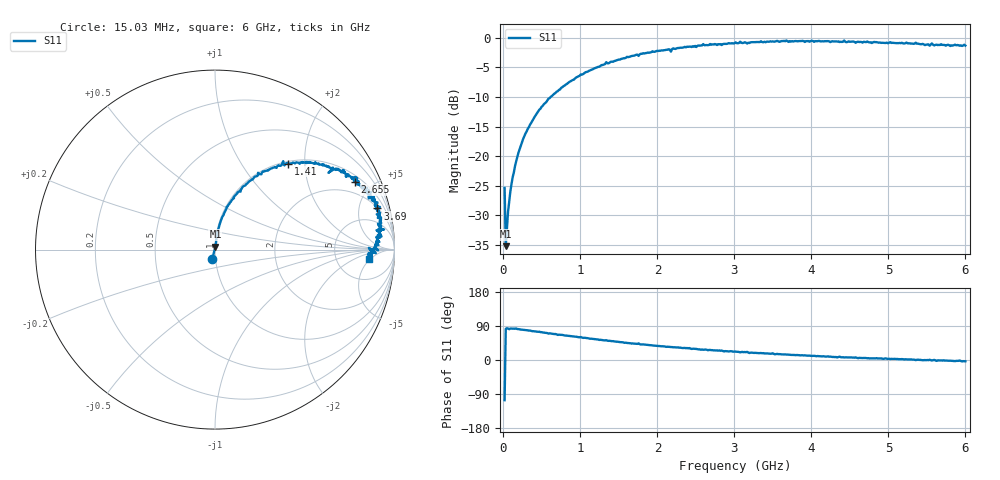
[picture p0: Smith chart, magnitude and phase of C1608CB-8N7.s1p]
!	Network	Analyzer	HP8753E.07.74:	Oct	30	2002	Serial	No.	JP38451487
!	Hewlett-Packard
!	28	Aug	2009	7:51:57
!	Frequency	S11
#	HZ	S	RI	R	50
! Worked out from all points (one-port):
!   400 points, 15.03 MHz to 6 GHz, reference 50 ohm
!   lowest |S11| = -35.2 dB at 30.03 MHz (marker M1), VSWR 1.04, Z = 50.2 + j1.73 ohm
!   |S11| at or under -10 dB: start of sweep to 613.1 MHz
!   S11 on the Smith chart (normalised r, x): 15.03 MHz: 0.97, -0.10; 1.41 GHz: 1.04, +1.65; 2.655 GHz: 1.31, +3.95; 3.69 GHz: 2.09, +7.45; 6 GHz: 12, -4
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1.502992e7  -0.0149 -0.0518
3.002985e7  0.00234 0.0172
6.00297e7  0.00416 0.0338
1.050295e8  0.00719 0.058
1.650292e8  0.0105 0.0897
2.550287e8  0.0249 0.137
4.650277e8  0.0651 0.238
7.650262e8  0.154 0.35
1.005025e9  0.24 0.428
1.410023e9  0.407 0.479
1.515022e9  0.445 0.48
2.265019e9  0.685 0.45
2.655017e9  0.779 0.377
3.015015e9  0.847 0.345
3.075015e9  0.87 0.318
3.165014e9  0.831 0.329
3.195014e9  0.857 0.285
3.495013e9  0.887 0.284
3.525012e9  0.896 0.239
3.690012e9  0.905 0.229
3.765011e9  0.904 0.221
4.335008e9  0.923 0.109
4.365008e9  0.909 0.142
4.425008e9  0.942 0.112
4.515007e9  0.92 0.111
5.265004e9  0.898 0.0215
5.535002e9  0.857 0.00958
6e9  0.858 -0.0501
